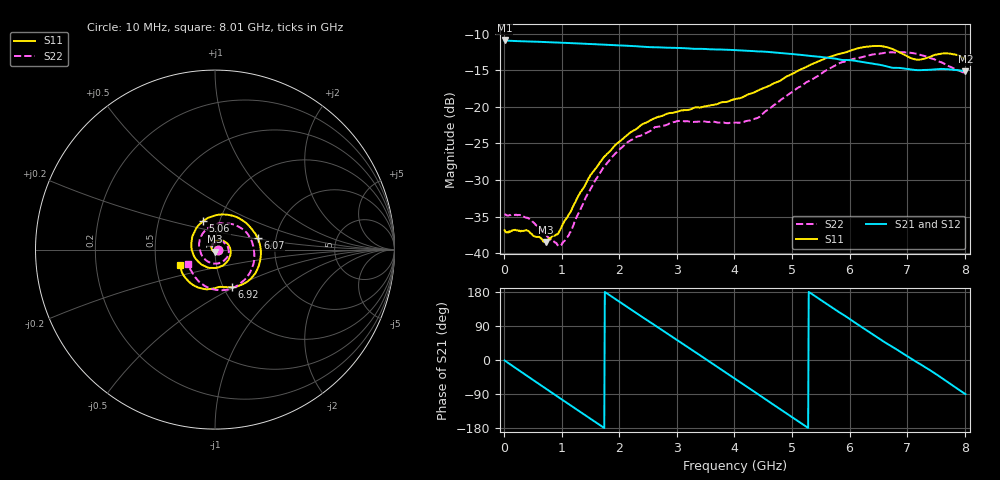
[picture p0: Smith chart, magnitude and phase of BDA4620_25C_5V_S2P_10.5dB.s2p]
!Agilent Technologies,E5071B,MY42404982,A.09.10
!Date: Wed May 06 09:00:21 2026
!Data & Calibration Information:
!Freq	S11:SOLT2(ON)	S21:SOLT2(ON)	S12:SOLT2(ON)	S22:SOLT2(ON)
# Hz S RI R 50
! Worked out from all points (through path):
!   801 points, 10 MHz to 8.01 GHz, reference 50 ohm
!   highest |S21| = -10.94 dB at 10 MHz (marker M1); lowest = -15.2 dB at 8.01 GHz (marker M2)
!   group delay of S21, straight-line fit = 281 ps
!   lowest |S11| = -38.5 dB at 720 MHz (marker M3), VSWR 1.02, Z = 49.8 - j1.18 ohm
!   |S11| at or under -10 dB: start of sweep to end of sweep
!   |S22| runs from -39.0 to -12.5 dB; largest |S21 - S12| = 0.0012
!   S11 on the Smith chart (normalised r, x): 10 MHz: 1.03, -0.00; 5.06 GHz: 0.84, +0.27; 6.07 GHz: 1.60, +0.22; 6.92 GHz: 1.09, -0.48; 8.01 GHz: 0.67, -0.12
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1e7  0.0143 -0.000953  0.2838 -0.00605  0.2841 -0.00615  0.0185 -0.0011
4.3e8  0.00977 -0.0102  0.1976 -0.1974  0.1979 -0.1979  0.0135 -0.0108
7.2e8  -0.00152 -0.0118  0.072 -0.2673  0.0719 -0.2678  0.00278 -0.0133
9.9e8  -0.014 -0.00481  -0.0603 -0.2673  -0.0607 -0.2678  -0.00906 -0.00686
1.35e9  -0.0201 0.0179  -0.2061 -0.1749  -0.2063 -0.175  -0.0159 0.0133
1.94e9  0.0173 0.0524  -0.2479 0.0891  -0.2482 0.0895  0.0133 0.0465
2.32e9  0.0583 0.0418  -0.1353 0.2205  -0.1356 0.221  0.0481 0.0403
2.68e9  0.0854 0.00306  0.0204 0.254  0.0206 0.2544  0.0719 0.0133
3e9  0.0806 -0.0451  0.1516 0.2021  0.152 0.2023  0.076 -0.0236
3.39e9  0.0372 -0.0916  0.2416 0.0591  0.2422 0.0588  0.0455 -0.0646
4.01e9  -0.0784 -0.081  0.1585 -0.1853  0.1586 -0.1857  -0.0472 -0.0621
4.51e9  -0.1324 0.0228  -0.0438 -0.2341  -0.0441 -0.2345  -0.0888 0.0204
5.06e9  -0.0655 0.1592  -0.2098 -0.0897  -0.2105 -0.0896  -0.0246 0.1289
5.35e9  0.023 0.1948  -0.2205 0.0244  -0.2208 0.0245  0.0486 0.146
5.67e9  0.1346 0.1745  -0.1681 0.135  -0.1681 0.1355  0.1339 0.1265
6.07e9  0.2374 0.0647  -0.0397 0.2028  -0.0395 0.2033  0.2102 0.0307
6.38e9  0.2506 -0.0668  0.0684 0.1855  0.0686 0.1857  0.2173 -0.0644
6.68e9  0.1794 -0.1793  0.1428 0.1206  0.1433 0.1208  0.1784 -0.153
6.92e9  0.0936 -0.2099  0.1746 0.0558  0.1749 0.0557  0.12 -0.2034
7.19e9  0.0282 -0.2074  0.1764 -0.0233  0.1769 -0.0234  0.0302 -0.227
7.57e9  -0.0815 -0.2148  0.1294 -0.1272  0.1298 -0.1273  -0.0799 -0.1858
8.01e9  -0.1934 -0.085  -0.000369 -0.1744  -0.000396 -0.1748  -0.148 -0.0798
